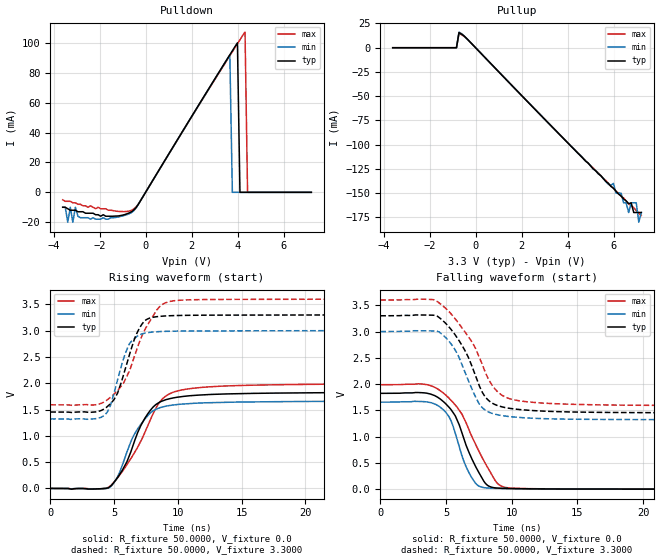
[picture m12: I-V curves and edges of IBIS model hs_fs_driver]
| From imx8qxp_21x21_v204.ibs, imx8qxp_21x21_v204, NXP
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[Model]  hs_fs_driver
|   Model hs_fs_driver
| This model was characterised for following simulation conditions:
| Spice Models:
|  - Typ Condition
|   /project/usb2_ln28fdsoi/HS/s2ibis/FS/ln28fdsoi_lp2.combination ln28fdsoi_typ
|  - Min Condition
|   /project/usb2_ln28fdsoi/HS/s2ibis/FS/ln28fdsoi_lp2.combination ln28fdsoi_wcs
|  - Max Condition
|   /project/usb2_ln28fdsoi/HS/s2ibis/FS/ln28fdsoi_lp2.combination ln28fdsoi_bcs
Model_type Output
Polarity   Non-Inverting
Enable   Active-Low
C_comp   2.8431pF   2.6338pF   3.0727pF
[Temperature Range]   27.0000   -40.0000   0.1050k
[Voltage Range]   3.3000V   3.0000V   3.6000V
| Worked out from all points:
|   slope of the pulldown table from 0 to 0.495 V, typ, clamps not added: 39.2 ohm
|   slope of the pullup table from 0 to 0.495 V, typ, clamps not added: 40.4 ohm
|   rising waveform, R_fixture 50.0000, V_fixture 0.0: 20-80 % time 2.07ns typ, 1.96ns min, 2.57ns max; typ from 0 V to 1.82 V
|   rising waveform, R_fixture 50.0000, V_fixture 3.3000: 20-80 % time 1.46ns typ, 1.23ns min, 2.15ns max; typ from 1.45 V to 3.3 V
|   falling waveform, R_fixture 50.0000, V_fixture 0.0: 20-80 % time 1.86ns typ, 1.37ns min, 2.46ns max; typ from 1.82 V to 0 V
|   falling waveform, R_fixture 50.0000, V_fixture 3.3000: 20-80 % time 2.1ns typ, 1.79ns min, 2.63ns max; typ from 3.3 V to 1.45 V
[Pulldown]
|Voltage   I(typ)   I(min)   I(max)
-3.6V     -10mA      -10mA      -5mA
-3.38V    -11mA      -20mA      -6mA
-3.27V    -12mA      -10mA      -6mA
-3.16V    -12mA      -20mA      -7mA
-520mV    -11.99mA   -12.49mA   -11.23mA
3.66V     92.06mA    91.98mA    91.46mA
3.77V     94.77mA    0A         94.14mA
3.99V     100.1mA    0A         99.47mA
4.1V      0A         0A         102.1mA
4.32V     0A         0A         107.3mA
4.43V     0A         0A         0A
7.2V      0A         0A         0A
[Pullup]
|Voltage   I(typ)   I(min)   I(max)
-3.6V     0A         0A         0A
-830mV    0A         0A         0A
-720mV    15.57mA    16.12mA    14.85mA
-610mV    14.08mA    14.52mA    13.43mA
5.77V     -140mA     -141mA     -140mA
5.99V     -145mA     -140mA     -145mA
6.32V     -153mA     -150mA     -153mA
6.65V     -161mA     -170mA     -161mA
6.76V     -160mA     -160mA     -163mA
6.98V     -170mA     -160mA     -168mA
7.09V     -170mA     -180mA     -171mA
7.2V      -170mA     -170mA     -173mA
[Ramp]
| variable   typ   min   max
dV/dt_r  1.0942/2.0703n   0.9938/1.9586n   1.1926/2.5668n
dV/dt_f  1.1082/2.0983n   1.0068/1.7883n   1.2059/2.6324n
R_load = 50.0000
[Rising Waveform]
R_fixture= 50.0000
V_fixture= 0.0
V_fixture_min= 0.0
V_fixture_max= 0.0
|time   V(typ)   V(min)   V(max)
0s        73.74nV    1.952nV    5.704uV
4.601ns   20.57mV    12.67mV    26.39mV
5.298ns   215.6mV    231.6mV    207.2mV
6.006ns   505.4mV    690.8mV    449.7mV
6.642ns   927.1mV    1.051V     697mV
7.512ns   1.371V     1.347V     1.121V
8.622ns   1.645V     1.536V     1.655V
9.92ns    1.732V     1.594V     1.85V
14.53ns   1.801V     1.641V     1.954V
30ns      1.824V     1.656V     1.988V
[Rising Waveform]
R_fixture= 50.0000
V_fixture= 3.3000
V_fixture_min= 3.0000
V_fixture_max= 3.6000
|time   V(typ)   V(min)   V(max)
0s        1.453V     1.322V     1.589V
3.687ns   1.46V      1.33V      1.595V
4.688ns   1.603V     1.564V     1.725V
5.276ns   1.812V     2.067V     1.862V
6.289ns   2.609V     2.778V     2.288V
6.75ns    2.93V      2.882V     2.621V
7.378ns   3.18V      2.95V      3V
8.536ns   3.27V      2.981V     3.448V
9.242ns   3.281V     2.987V     3.547V
30ns      3.3V       3V         3.6V
[Falling Waveform]
R_fixture= 50.0000
V_fixture= 0.0
V_fixture_min= 0.0
V_fixture_max= 0.0
|time   V(typ)   V(min)   V(max)
0s        1.824V     1.656V     1.988V
3.346ns   1.833V     1.665V     1.997V
4.738ns   1.681V     1.525V     1.843V
5.189ns   1.571V     1.397V     1.743V
5.701ns   1.399V     1.069V     1.603V
6.402ns   923.7mV    504.4mV    1.332V
7.207ns   453.9mV    126.6mV    876.3mV
8.13ns    79.07mV    22.41mV    428.7mV
9.414ns   14.79mV    11.12mV    40.18mV
30ns      229.7uV    166.1uV    352.6uV
[Falling Waveform]
R_fixture= 50.0000
V_fixture= 3.3000
V_fixture_min= 3.0000
V_fixture_max= 3.6000
|time   V(typ)   V(min)   V(max)
0s        3.3V       3V         3.6V
4.349ns   3.291V     3.004V     3.569V
5.384ns   3.041V     2.768V     3.337V
6.21ns    2.741V     2.372V     3.074V
7.211ns   2.181V     1.775V     2.699V
7.707ns   1.872V     1.566V     2.405V
8.771ns   1.606V     1.425V     1.894V
10.16ns   1.527V     1.373V     1.7V
15.8ns    1.464V     1.329V     1.608V
30ns      1.453V     1.322V     1.59V
